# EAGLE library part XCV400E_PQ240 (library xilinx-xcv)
xcv400e_pq240 edit this description Auto generated by make-symbol-device-package-bsdl.ulp Rev. 26 Source: xcv400e_pq240.bsd
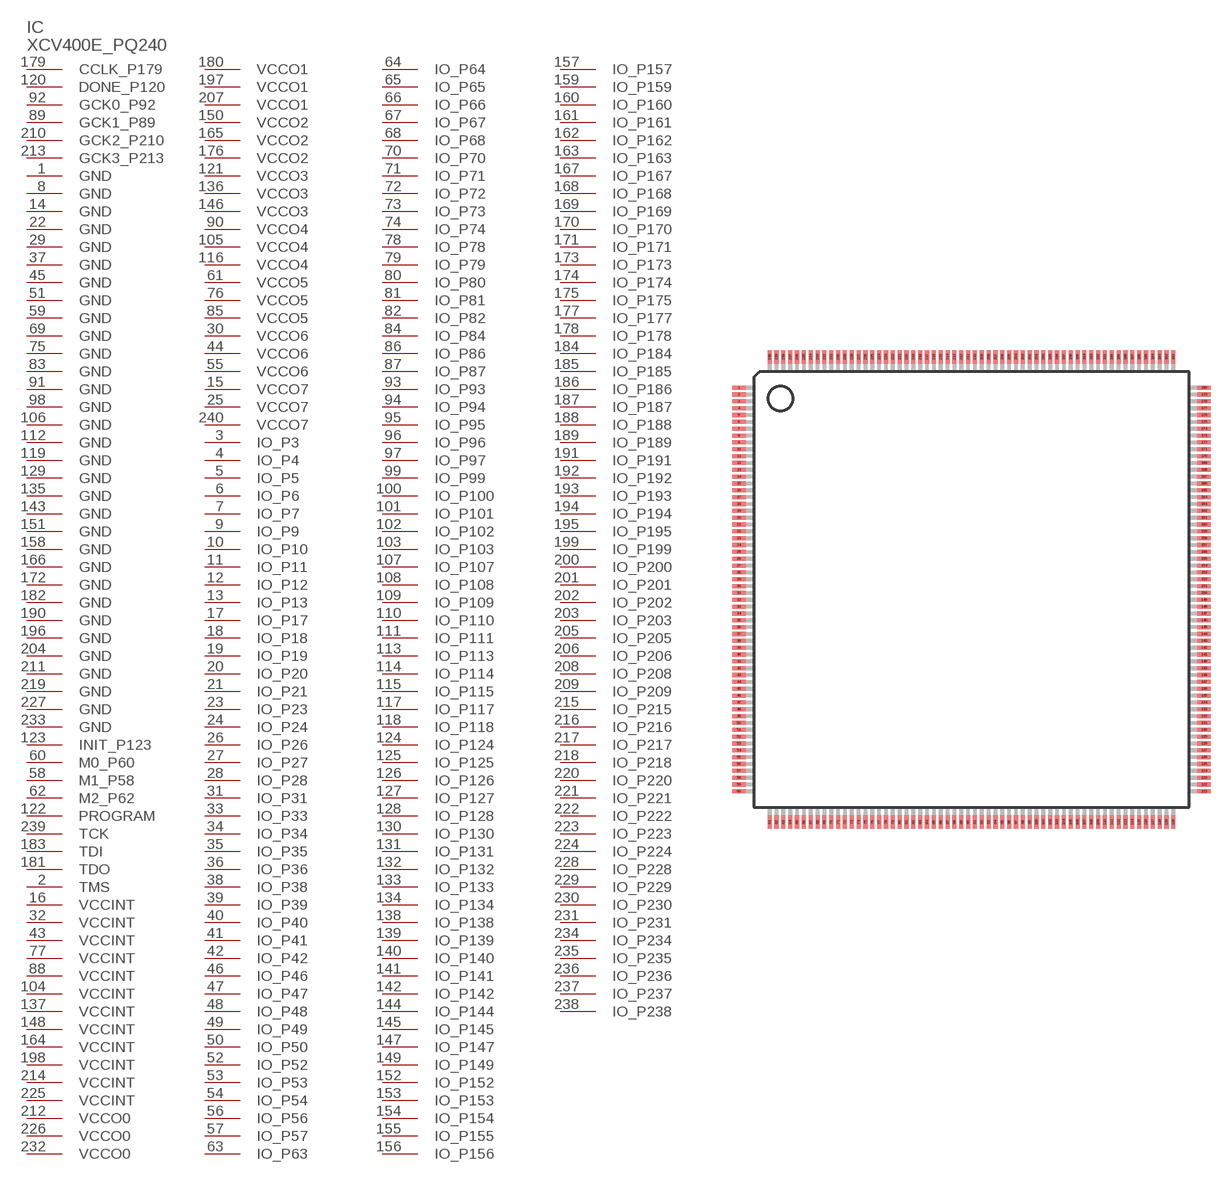
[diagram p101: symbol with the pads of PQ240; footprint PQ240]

Designator prefix IC

## XCV400E_PQ240 (OC_FARNELL: unknown; OC_NEWARK: unknown)  [PQ240]
1  GND  pwr
2  TMS  in
3  IO_P3
4  IO_P4
5  IO_P5
6  IO_P6
7  IO_P7
8  GND  pwr
9  IO_P9
10  IO_P10
11  IO_P11
12  IO_P12
13  IO_P13
14  GND  pwr
15  VCCO7  pwr
16  VCCINT  pwr
17  IO_P17
18  IO_P18
19  IO_P19
20  IO_P20
21  IO_P21
22  GND  pwr
23  IO_P23
24  IO_P24
25  VCCO7  pwr
26  IO_P26
27  IO_P27
28  IO_P28
29  GND  pwr
30  VCCO6  pwr
31  IO_P31
32  VCCINT  pwr
33  IO_P33
34  IO_P34
35  IO_P35
36  IO_P36
37  GND  pwr
38  IO_P38
39  IO_P39
40  IO_P40
41  IO_P41
42  IO_P42
43  VCCINT  pwr
44  VCCO6  pwr
45  GND  pwr
46  IO_P46
47  IO_P47
48  IO_P48
49  IO_P49
50  IO_P50
51  GND  pwr
52  IO_P52
53  IO_P53
54  IO_P54
55  VCCO6  pwr
56  IO_P56
57  IO_P57
58  M1_P58  in
59  GND  pwr
60  M0_P60  in
61  VCCO5  pwr
62  M2_P62  in
63  IO_P63
64  IO_P64
65  IO_P65
66  IO_P66
67  IO_P67
68  IO_P68
69  GND  pwr
70  IO_P70
71  IO_P71
72  IO_P72
73  IO_P73
74  IO_P74
75  GND  pwr
76  VCCO5  pwr
77  VCCINT  pwr
78  IO_P78
79  IO_P79
80  IO_P80
81  IO_P81
82  IO_P82
83  GND  pwr
84  IO_P84
85  VCCO5  pwr
86  IO_P86
87  IO_P87
88  VCCINT  pwr
89  GCK1_P89  in
90  VCCO4  pwr
91  GND  pwr
92  GCK0_P92  in
93  IO_P93
94  IO_P94
95  IO_P95
96  IO_P96
97  IO_P97
98  GND  pwr
99  IO_P99
100  IO_P100
101  IO_P101
102  IO_P102
103  IO_P103
104  VCCINT  pwr
105  VCCO4  pwr
106  GND  pwr
107  IO_P107
108  IO_P108
109  IO_P109
110  IO_P110
111  IO_P111
112  GND  pwr
113  IO_P113
114  IO_P114
115  IO_P115
116  VCCO4  pwr
117  IO_P117
118  IO_P118
119  GND  pwr
120  DONE_P120
121  VCCO3  pwr
122  PROGRAM  in
123  INIT_P123
124  IO_P124
125  IO_P125
126  IO_P126
127  IO_P127
128  IO_P128
129  GND  pwr
130  IO_P130
131  IO_P131
132  IO_P132
133  IO_P133
134  IO_P134
135  GND  pwr
136  VCCO3  pwr
137  VCCINT  pwr
138  IO_P138
139  IO_P139
140  IO_P140
141  IO_P141
142  IO_P142
143  GND  pwr
144  IO_P144
145  IO_P145
146  VCCO3  pwr
147  IO_P147
148  VCCINT  pwr
149  IO_P149
150  VCCO2  pwr
151  GND  pwr
152  IO_P152
153  IO_P153
154  IO_P154
155  IO_P155
156  IO_P156
157  IO_P157
158  GND  pwr
159  IO_P159
160  IO_P160
161  IO_P161
162  IO_P162
163  IO_P163
164  VCCINT  pwr
165  VCCO2  pwr
166  GND  pwr
167  IO_P167
168  IO_P168
169  IO_P169
170  IO_P170
171  IO_P171
172  GND  pwr
173  IO_P173
174  IO_P174
175  IO_P175
176  VCCO2  pwr
177  IO_P177
178  IO_P178
179  CCLK_P179
180  VCCO1  pwr
181  TDO  out
182  GND  pwr
183  TDI  in
184  IO_P184
185  IO_P185
186  IO_P186
187  IO_P187
188  IO_P188
189  IO_P189
190  GND  pwr
191  IO_P191
192  IO_P192
193  IO_P193
194  IO_P194
195  IO_P195
196  GND  pwr
197  VCCO1  pwr
198  VCCINT  pwr
199  IO_P199
200  IO_P200
201  IO_P201
202  IO_P202
203  IO_P203
204  GND  pwr
205  IO_P205
206  IO_P206
207  VCCO1  pwr
208  IO_P208
209  IO_P209
210  GCK2_P210  in
211  GND  pwr
212  VCCO0  pwr
213  GCK3_P213  in
214  VCCINT  pwr
215  IO_P215
216  IO_P216
217  IO_P217
218  IO_P218
219  GND  pwr
220  IO_P220
221  IO_P221
222  IO_P222
223  IO_P223
224  IO_P224
225  VCCINT  pwr
226  VCCO0  pwr
227  GND  pwr
228  IO_P228
229  IO_P229
230  IO_P230
231  IO_P231
232  VCCO0  pwr
233  GND  pwr
234  IO_P234
235  IO_P235
236  IO_P236
237  IO_P237
238  IO_P238
239  TCK  in
240  VCCO7  pwr

## Footprint PQ240 (pad centres in mm)
PQ240 Auto generated by make-symbol-device-package-bsdl.ulp Rev. 26
smd 1 x 0.3: 1 -17,14.75; 2 -17,14.25; 3 -17,13.75; 4 -17,13.25; 5 -17,12.75; 6 -17,12.25; 7 -17,11.75; 8 -17,11.25; 9 -17,10.75; 10 -17,10.25; 11 -17,9.75; 12 -17,9.25; 13 -17,8.75; 14 -17,8.25; 15 -17,7.75; 16 -17,7.25; 17 -17,6.75; 18 -17,6.25; 19 -17,5.75; 20 -17,5.25; 21 -17,4.75; 22 -17,4.25; 23 -17,3.75; 24 -17,3.25; 25 -17,2.75; 26 -17,2.25; 27 -17,1.75; 28 -17,1.25; 29 -17,0.75; 30 -17,0.25; 31 -17,-0.25; 32 -17,-0.75; 33 -17,-1.25; 34 -17,-1.75; 35 -17,-2.25; 36 -17,-2.75; 37 -17,-3.25; 38 -17,-3.75; 39 -17,-4.25; 40 -17,-4.75; 41 -17,-5.25; 42 -17,-5.75; 43 -17,-6.25; 44 -17,-6.75; 45 -17,-7.25; 46 -17,-7.75; 47 -17,-8.25; 48 -17,-8.75; 49 -17,-9.25; 50 -17,-9.75; 51 -17,-10.25; 52 -17,-10.75; 53 -17,-11.25; 54 -17,-11.75; 55 -17,-12.25; 56 -17,-12.75; 57 -17,-13.25; 58 -17,-13.75; 59 -17,-14.25; 60 -17,-14.75; 121 17,-14.75; 122 17,-14.25; 123 17,-13.75; 124 17,-13.25; 125 17,-12.75; 126 17,-12.25; 127 17,-11.75; 128 17,-11.25; 129 17,-10.75; 130 17,-10.25; 131 17,-9.75; 132 17,-9.25; 133 17,-8.75; 134 17,-8.25; 135 17,-7.75; 136 17,-7.25; 137 17,-6.75; 138 17,-6.25; 139 17,-5.75; 140 17,-5.25; 141 17,-4.75; 142 17,-4.25; 143 17,-3.75; 144 17,-3.25; 145 17,-2.75; 146 17,-2.25; 147 17,-1.75; 148 17,-1.25; 149 17,-0.75; 150 17,-0.25; 151 17,0.25; 152 17,0.75; 153 17,1.25; 154 17,1.75; 155 17,2.25; 156 17,2.75; 157 17,3.25; 158 17,3.75; 159 17,4.25; 160 17,4.75; 161 17,5.25; 162 17,5.75; 163 17,6.25; 164 17,6.75; 165 17,7.25; 166 17,7.75; 167 17,8.25; 168 17,8.75; 169 17,9.25; 170 17,9.75; 171 17,10.25; 172 17,10.75; 173 17,11.25; 174 17,11.75; 175 17,12.25; 176 17,12.75; 177 17,13.25; 178 17,13.75; 179 17,14.25; 180 17,14.75
smd 0.3 x 1: 61 -14.75,-17; 62 -14.25,-17; 63 -13.75,-17; 64 -13.25,-17; 65 -12.75,-17; 66 -12.25,-17; 67 -11.75,-17; 68 -11.25,-17; 69 -10.75,-17; 70 -10.25,-17; 71 -9.75,-17; 72 -9.25,-17; 73 -8.75,-17; 74 -8.25,-17; 75 -7.75,-17; 76 -7.25,-17; 77 -6.75,-17; 78 -6.25,-17; 79 -5.75,-17; 80 -5.25,-17; 81 -4.75,-17; 82 -4.25,-17; 83 -3.75,-17; 84 -3.25,-17; 85 -2.75,-17; 86 -2.25,-17; 87 -1.75,-17; 88 -1.25,-17; 89 -0.75,-17; 90 -0.25,-17; 91 0.25,-17; 92 0.75,-17; 93 1.25,-17; 94 1.75,-17; 95 2.25,-17; 96 2.75,-17; 97 3.25,-17; 98 3.75,-17; 99 4.25,-17; 100 4.75,-17; 101 5.25,-17; 102 5.75,-17; 103 6.25,-17; 104 6.75,-17; 105 7.25,-17; 106 7.75,-17; 107 8.25,-17; 108 8.75,-17; 109 9.25,-17; 110 9.75,-17; 111 10.25,-17; 112 10.75,-17; 113 11.25,-17; 114 11.75,-17; 115 12.25,-17; 116 12.75,-17; 117 13.25,-17; 118 13.75,-17; 119 14.25,-17; 120 14.75,-17; 181 14.75,17; 182 14.25,17; 183 13.75,17; 184 13.25,17; 185 12.75,17; 186 12.25,17; 187 11.75,17; 188 11.25,17; 189 10.75,17; 190 10.25,17; 191 9.75,17; 192 9.25,17; 193 8.75,17; 194 8.25,17; 195 7.75,17; 196 7.25,17; 197 6.75,17; 198 6.25,17; 199 5.75,17; 200 5.25,17; 201 4.75,17; 202 4.25,17; 203 3.75,17; 204 3.25,17; 205 2.75,17; 206 2.25,17; 207 1.75,17; 208 1.25,17; 209 0.75,17; 210 0.25,17; 211 -0.25,17; 212 -0.75,17; 213 -1.25,17; 214 -1.75,17; 215 -2.25,17; 216 -2.75,17; 217 -3.25,17; 218 -3.75,17; 219 -4.25,17; 220 -4.75,17; 221 -5.25,17; 222 -5.75,17; 223 -6.25,17; 224 -6.75,17; 225 -7.25,17; 226 -7.75,17; 227 -8.25,17; 228 -8.75,17; 229 -9.25,17; 230 -9.75,17; 231 -10.25,17; 232 -10.75,17; 233 -11.25,17; 234 -11.75,17; 235 -12.25,17; 236 -12.75,17; 237 -13.25,17; 238 -13.75,17; 239 -14.25,17; 240 -14.75,17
